(* Logix 5000 AddOnInstructionDefinition export MHSI_Yaskawa; software revision 17.00 *)

TYPE Yaskawa_EIP_Servo :   // Yaskawa SigmaLogic Axis Structure v2.4.0
STRUCT
   O : Yaskawa_OUT_to_Servo;
   I : Yaskawa_IN_from_Servo;
   AOI_SB : Yaskawa_AOI_Status_Bits;
END_STRUCT
END_TYPE

TYPE Yaskawa_OUT_to_Servo :   // Structure of data sent out to the Yaskawa SigmaLogic controller v2.4.0
STRUCT
   b00_ServoOn : BOOL;   // Servo On
   b01_Stop : BOOL;   // Stops All Current Motion in Progress
   b02_Home : BOOL;   // Start Homing Process
   b03_MoveStart1 : BOOL;   // Start Current Motion
   b06_SuperImpose : BOOL;
   b07_ServoAlarmReset : BOOL;   // Servo Alarm Reset
   b08_ControllerAlarmReset : BOOL;   // SigmaLogic Alarm Reset
   b09_MoveStart2 : BOOL;   // Start Second Motion (Blended Move)
   b10_MoveAbort : BOOL;   // Abort Current Move
   b11_MovePause : BOOL;   // Pause Current Move
   b12_SeqPause : BOOL;   // Indexing Sequence Pause
   b13_SeqResume : BOOL;   // Indexing Sequence Resume
   b14_SeqCancel : BOOL;   // Indexing Sequence Cancel
   b15_AbsEncoderReset : BOOL;   // Absolute Encoder Reset
   b16_SeqStart : BOOL;   // Start Indexing Sequence
   b17_SeqEditSpeed : BOOL;   // Enter Edit Speed
   b18_SeqEditDistance : BOOL;   // Enter Distance Edit
   b19_PLSEnable : BOOL;   // Enable PLS execution
   b20_PLSActivateOutput1 : BOOL;   // Activate PLS output1 switch logic
   b21_PLSActivateOutput2 : BOOL;   // Activate PLS output2 switch logic
   b22_PLSActivateOutput3 : BOOL;   // Activate PLS output3 switch logic
   b23_PLSActivateOutput4 : BOOL;   // Activate PLS output4 switch logic
   b24_SetClock : BOOL;   // Set the remote controller clock with data provided by the PLC
   RebootController : BOOL;
   UseExternalEncoder : BOOL;   // Use External Encoder when executing MAHSP_Yaskawa
   b32_HeatbeatAnswer : BOOL;   // Heartbeat Answer
   BrakeBypassRequest : BOOL;
   SetFwdTorqueLimit : BOOL;
   SetRevTorqueLimit : BOOL;
   TorqueLimit : DINT;
   TorqueRamp : DINT;
   HomeMethod : INT;
   HomeSpeed : DINT;
   HomeAccDec : DINT;   // Home Move Acceleration/Deceleration Rate
   HomeBackOffDistance : DINT;
   HomeCreepSpeed : DINT;
   HomeCreepDistanceLimit : DINT;
   HomeCreepTimeLimit : DINT;
   HomeOffsetDistance : DINT;
   HomeOffsetSpeed : DINT;
   HomePostion : DINT;
   HomeTorque : DINT;
   HomeInputNo : DINT;
   HomeApproachTimeLimit : DINT;
   HomeApproachDistLimit : DINT;
   HomeDirection : INT;
   HomeSwitchMode : INT;
   MoveType : INT;
   MoveDirection : INT;
   MoveAccel1 : DINT;
   MoveAccel2 : DINT;
   MoveDecel1 : DINT;
   MoveDecel2 : DINT;
   MoveSpeed1 : DINT;
   MoveSpeed2 : DINT;
   MoveDistance1 : DINT;
   MoveDistance2 : DINT;
   MovePosition1 : DINT;
   MovePosition2 : DINT;
   RegistrationDistance : DINT;
   GearNumerator : DINT;
   GearDenominator : DINT;
   SuperImposeDistance : DINT;
   Resolution : INT;
   RegistrationDirection : INT;
   TuningLevel : INT;
   SequenceStep : INT;   // Staring Sequence Step Number
   SequenceEditStep : INT;   // Sequence Step Number to Edit
   FlagCommandBits1 : DINT;   // Flag Commands. 1..64 are General Flags, Bits 0..31 correspond to Flag 1..32
   FlagCommandBits2 : DINT;   // Flag Commands cont. 1..64 are General Flags, Bits 0..31 correspond to Flag 33..64
   DigitalOutCommandBits : DINT;   // Digital Output commands. Bits 0-7 correspond to CN13 Digital Outputs 0-7, used as Flag 73-80. Bits 8-10 correspond to CN1 Digital Outputs 0-2 used as Flag 88-90"
   SequenceEditSpeed : DINT;
   SequenceEditDistance : DINT;
   FeedRateOverride : INT;
   HSI_Enable : BOOL;
   HSI_MoveMode : BOOL;   // 0=Relative; 1=Moves per Cycle
   HSI_CalcMethod : BOOL;   // 0=Accel/Decel; 1=Time
   HSI_MoveDirection : BOOL;   // 0 = Negative; 1 = Positive
   HSI_TriggerFlag : INT;
   HSI_MovingFlag : INT;
   HSI_DwellingFlag : INT;
   HSI_DoneFlag : INT;
   HSI_MoveType : INT;   // 0=Single; 1=Repeat; 2=Repeat "x" times
   HSI_RepeatNumber : INT;
   HSI_Distance : DINT;
   HSI_Speed : DINT;
   HSI_Accel : DINT;
   HSI_MoveTime : DINT;
   HSI_DwellTime : DINT;
   PLS_OutputFlag1 : INT;
   PLS_OutputFlag2 : INT;
   PLS_OutputFlag3 : INT;
   PLS_OutputFlag4 : INT;
   PLS_OnPosition1 : DINT;
   PLS_OffPosition1 : DINT;
   PLS_OnPosition2 : DINT;
   PLS_OffPosition2 : DINT;
   PLS_OnPosition3 : DINT;
   PLS_OffPosition3 : DINT;
   PLS_OnPosition4 : DINT;
   PLS_OffPosition4 : DINT;
   PLS_OnCompensation1 : INT;
   PLS_OffCompensation1 : INT;
   PLS_OnCompensation2 : INT;
   PLS_OffCompensation2 : INT;
   PLS_OnCompensation3 : INT;
   PLS_OffCompensation3 : INT;
   PLS_OnCompensation4 : INT;
   PLS_OffCompensation4 : INT;
   RTC_Year : INT;
   RTC_Month : INT;
   RTC_Day : INT;
   RTC_Hour : INT;
   RTC_Min : INT;
   RTC_Sec : INT;
   StopDecel : DINT;
   AnalogOutput : INT;   // CN13, AO_01 [mV]
END_STRUCT
END_TYPE

TYPE Yaskawa_AOI_Status_Bits :   // Internal bits used to interlock Yaskawa AOI execution. v2.4.0
STRUCT
   MAM : BOOL;   // Move AOI Active
   MAJ : BOOL;   // Jog AOI Active
   MAB : BOOL;   // Blending AOI Active
   MAG : BOOL;   // Gearing AOI Active
   MAHSP : BOOL;   // Home SetPoint AOI Active
   MAH : BOOL;   // Homing AOI Active
   MSQE : BOOL;   // Sequence Edit AOI Active
   MSQR : BOOL;   // Sequence Run AOI Active
   MHSI : BOOL;   // High Speed Index AOI Active
   MSO : BOOL;   // Servo On
   MSF : BOOL;   // Servo Off
   MAFR : BOOL;   // Fault Reset
   MAS : BOOL;   // Servo Abort
   MTRQ : BOOL;   // Torque Mode Active
   MPLS : BOOL;   // PLS Active
   MCLK : BOOL;   // SetClock Active
   MSTL : BOOL;   // Set Torque Limit Active
   AOI_Permissive : BOOL;   // Permissive to Execute an AOI
END_STRUCT
END_TYPE

TYPE Yaskawa_IN_from_Servo :   // Structure of data coming from the Yaskawa SigmaLogic controller. v2.4.0
STRUCT
   AlarmText : STRING;   // ServoPack Alarm Code plus Text Description
   b00_Heartbeat : BOOL;
   b01_Alarm : BOOL;   // ServoPack Alarm
   b02_Warning : BOOL;   // ServoPack Warning
   b03_Ready : BOOL;   // ServoPack Ready
   b04_Enabled : BOOL;   // ServoPack Enabled ("Servo On")
   b05_StopComplete : BOOL;
   b06_HomeComplete : BOOL;
   b07_HomeBusy : BOOL;
   b08_HomeActive : BOOL;
   b09_HomeAborted : BOOL;
   b10_HomeError : BOOL;
   b11_MoveAbsComplete : BOOL;
   b12_MoveAbsBusy : BOOL;
   b13_MoveAbsActive : BOOL;
   b14_MoveAbsAborted : BOOL;
   b15_MoveAbsError : BOOL;
   b16_MoveRelComplete : BOOL;
   b17_MoveRelBusy : BOOL;
   b18_MoveRelActive : BOOL;
   b19_MoveRelAborted : BOOL;
   b20_MoveRelError : BOOL;
   b21_JogAtSpeed : BOOL;
   b22_JogBusy : BOOL;
   b23_JogActive : BOOL;
   b24_JogAborted : BOOL;
   b25_JogError : BOOL;
   b26_GearInSync : BOOL;
   b27_GearBusy : BOOL;
   b28_GearActive : BOOL;
   b29_GearAborted : BOOL;
   b30_GearError : BOOL;
   b32_MoveSuperComplete : BOOL;
   b33_MoveSuperBusy : BOOL;
   b34_MoveSuperActive : BOOL;
   b35_MoveSuperAborted : BOOL;
   b36_MoveSuperError : BOOL;
   b37_PowerCycleRequired : BOOL;
   b38_MoveBlend1Complete : BOOL;
   b39_MoveBlend1Busy : BOOL;
   b40_MoveBlend1Active : BOOL;
   b41_MoveBlend1Abort : BOOL;
   b42_MoveBlend1Error : BOOL;
   b43_MoveBlend2Complete : BOOL;
   b44_MoveBlend2Busy : BOOL;
   b45_MoveBlend2Active : BOOL;
   b46_MoveBlend2Abort : BOOL;
   b47_MoveBlend2Error : BOOL;
   b48_RegComplete : BOOL;
   b49_RegBusy : BOOL;
   b50_RegActive : BOOL;
   b51_RegAborted : BOOL;
   b52_RegError : BOOL;
   b53_ResetAbsEncoderActive : BOOL;
   b54_ResetAbsEncoderBusy : BOOL;
   b55_ResetAbsEncoderDone : BOOL;
   b56_ResetAbsEncoderError : BOOL;
   b57_SeqRunning : BOOL;
   b58_RegSensorNotReached : BOOL;
   b59_SeqEditError : BOOL;
   b60_SeqEditDone : BOOL;
   b61_TorqueAtTorque : BOOL;
   b62_TorqueBusy : BOOL;
   b63_TorqueActive : BOOL;
   b64_TorqueAborted : BOOL;
   b65_TorqueError : BOOL;
   b66_ControllerAlarm : BOOL;
   b67_ApplicationError : BOOL;
   b68_AxisAtStandStill : BOOL;
   b69_TestModeActive : BOOL;
   b70_ServoParamsOK : BOOL;
   b71_SetFwdTorqueLimitDone : BOOL;
   b72_SetRevTorqueLimitDone : BOOL;
   Position : DINT;
   Speed : DINT;
   Torque : DINT;
   HomeErrorID : INT;
   MoveAbsErrorID : INT;
   MoveRelErrorID : INT;
   JogErrorID : INT;
   GearErrorID : INT;
   MoveSuperErrorID : INT;
   ServoAlarmID : INT;
   ServoWarningID : INT;
   ControllerAlarmID : DINT;
   AxisGenAlarmID : DINT;
   MoveBlend1ErrorID : INT;
   MoveBlend2ErrorID : INT;
   ResetAbsEncoderErrorID : INT;
   FunctionBlockErrorID : INT;
   TorqueErrorID : INT;
   RegErrorID : INT;
   SeqCurrentStep : INT;
   FlagStatusBit1 : DINT;   // Flag Status. 1..64 are General Flags, Bits 0..31 correspond to Flag 1..32
   FlagStatusBit2 : DINT;   // Flag Status cont. 1..64 are General Flags, Bits 0..31 correspond to Flag 33..64
   IOStatusBits : DINT;   // Digital IO Status. Bits 0-7, CN13 Inputs 0-7, Used as Flag 65-72. Bits 8-15, CN13 Outputs 0-7, Used as Flag 73-80. Bits 16-22, CN1 Inputs 0-6, Used as Flag 81-87. Bits 23-25, CN1 Outputs 0-4, Used as Flag 88-92.
   HSI_Moving : BOOL;
   HSI_Dwelling : BOOL;
   HSI_Done : BOOL;
   HSI_Busy : BOOL;
   HSI_Error : BOOL;
   HSI_ErrorCode : INT;
   PLS_Running : BOOL;
   PLS_SwitchStatus1 : BOOL;
   PLS_SwitchStatus2 : BOOL;
   PLS_SwitchStatus3 : BOOL;
   PLS_SwitchStatus4 : BOOL;
   PLS_Busy : BOOL;
   PLS_Error : BOOL;
   PLS_ErrorCode : INT;
   SetClock_Done : BOOL;
   SetClock_Busy : BOOL;
   SetClock_Error : BOOL;
   SetClock_ErrorID : INT;
   SoftwareVersion : DINT;
   FirmwareVersion : DINT;
   CommandedPos : DINT;
   CommandedPosNonCyc : DINT;
   CommandedSpeed : DINT;
   Clock_Year : INT;
   Clock_Month : INT;
   Clock_Day : INT;
   Clock_Hour : INT;
   Clock_Minute : INT;
   Clock_Second : INT;
   AnalogInput : REAL;   // CN13, AI_01 [v]
   BrakeBypassActive : BOOL;
   ForwardTorqueLimit : DINT;
   ReverseTorqueLimit : DINT;
END_STRUCT
END_TYPE

ADD_ON_INSTRUCTION MHSI_Yaskawa   (* revision 2.4 0, vendor Yaskawa America, Inc., ExecuteEnableInFalse *)
// Motion Axis High Speed Index
// Revision note:
// 2.4.0: No functional change
// 2.3.1: Moved unlatch of AOI_ON_LOCAL to bottom of EnableInFalse routine so that outputs will be on for at least 1 scan if one-shot on EN is used.
// 2.3.0: No functional change
// 2.0.0: Improved output operation and error code reporting. Improved interlocking with embedded code.
// 1.2.0: No functional change.
// Initial Release 9/10/2014
// Help:
// This AOI transfers settings to the remote axis node for high response motion to be executed in the remote node using local servo I/O. The motion goes through a Move-Dwell cycle when triggered. Move time can either be entered directly or derived from the Speed, Accel and Distance parameters.
VAR_IN_OUT
   Axis : Yaskawa_EIP_Servo; {required}
END_VAR
VAR_INPUT
   MoveMode : INT; {required}   // 0 = Relative 1 = Moves per Machine Cycle
   MoveType : INT; {required}   // 0 = Single 1 = Repeating Move 2 = Repeat for "x" Times
   RepeatNumber : INT; {required}   // For MoveType #2
   CalcMethod : INT; {required}   // 0 = Use Acc/ Decel 1 = Use Time
   Distance : REAL; {required}   // [units]
   Speed : REAL; {required}   // [units/s]
   Accel : REAL; {required}   // [units/s/s]
   MoveTime : DINT; {required}   // msec
   DwellTime : DINT; {required}   // msec
   Direction : INT; {required}   // 0 = Positive 1 = Negative
   TriggerFlagAssign : INT; {required}
   MovingFlagAssign : INT; {required}
   DwellingFlagAssign : INT; {required}
   DoneFlagAssign : INT; {required}
END_VAR
VAR_OUTPUT
   EN : BOOL; {visible}   // AOI is Active
   DN : BOOL; {visible}   // HSI Cycle (Index then Dwell) Completed
   IP : BOOL; {visible}   // HSI Busy (move in operation)
   ER : BOOL; {visible}   // HSI Error
   MV : BOOL; {visible}   // HSI Move (move is in motion)
   DW : BOOL; {visible}   // HSI Dwelling
   FLT_RDY : BOOL; {visible}   // The Servo is Not Ready
   FLT_BSY : BOOL; {visible}   // There is another AOI Active for this Axis
   ErrorCode : INT; {visible}   // ErrorID for High Speed Index function
END_VAR
VAR
   AOI_ON_LOCAL : BOOL;
   ScaleFactor : DINT;
   Finished : BOOL;   // Function is Finished
END_VAR

ROUTINE EnableInFalse   (* ladder *)
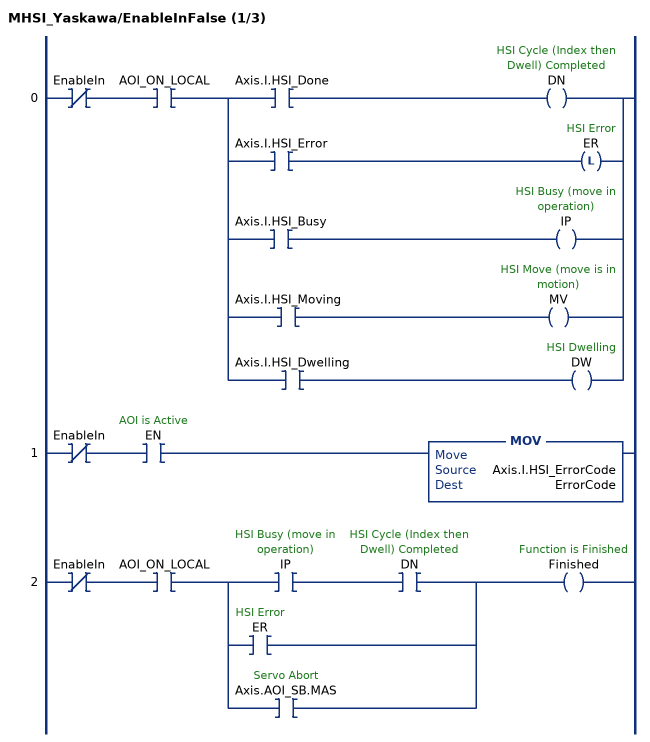
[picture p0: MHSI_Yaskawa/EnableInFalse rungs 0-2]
   0: XIO(EnableIn)XIC(AOI_ON_LOCAL)[XIC(Axis.I.HSI_Done) OTE(DN) ,XIC(Axis.I.HSI_Error) OTL(ER) ,XIC(Axis.I.HSI_Busy) OTE(IP) ,XIC(Axis.I.HSI_Moving) OTE(MV) ,XIC(Axis.I.HSI_Dwelling) OTE(DW) ];
   1: XIO(EnableIn)XIC(EN)MOV(Axis.I.HSI_ErrorCode,ErrorCode);
   2: XIO(EnableIn)XIC(AOI_ON_LOCAL)[XIC(IP) XIC(DN) ,XIC(ER) ,XIC(Axis.AOI_SB.MAS) ]OTE(Finished);
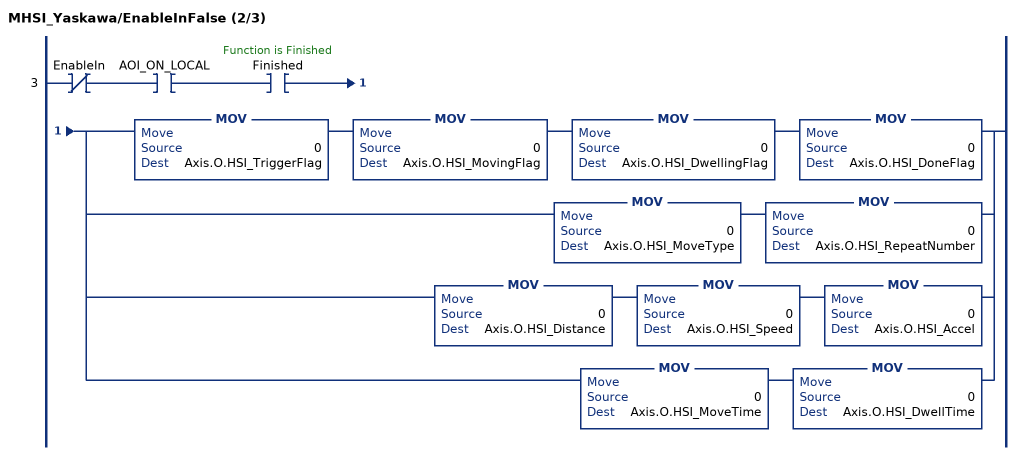
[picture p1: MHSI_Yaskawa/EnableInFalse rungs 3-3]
   3: XIO(EnableIn)XIC(AOI_ON_LOCAL)XIC(Finished)[MOV(0,Axis.O.HSI_TriggerFlag) MOV(0,Axis.O.HSI_MovingFlag) MOV(0,Axis.O.HSI_DwellingFlag) MOV(0,Axis.O.HSI_DoneFlag) ,MOV(0,Axis.O.HSI_MoveType) MOV(0,Axis.O.HSI_RepeatNumber) ,MOV(0,Axis.O.HSI_Distance) MOV(0,Axis.O.HSI_Speed) MOV(0,Axis.O.HSI_Accel) ,MOV(0,Axis.O.HSI_MoveTime) MOV(0,Axis.O.HSI_DwellTime) ];
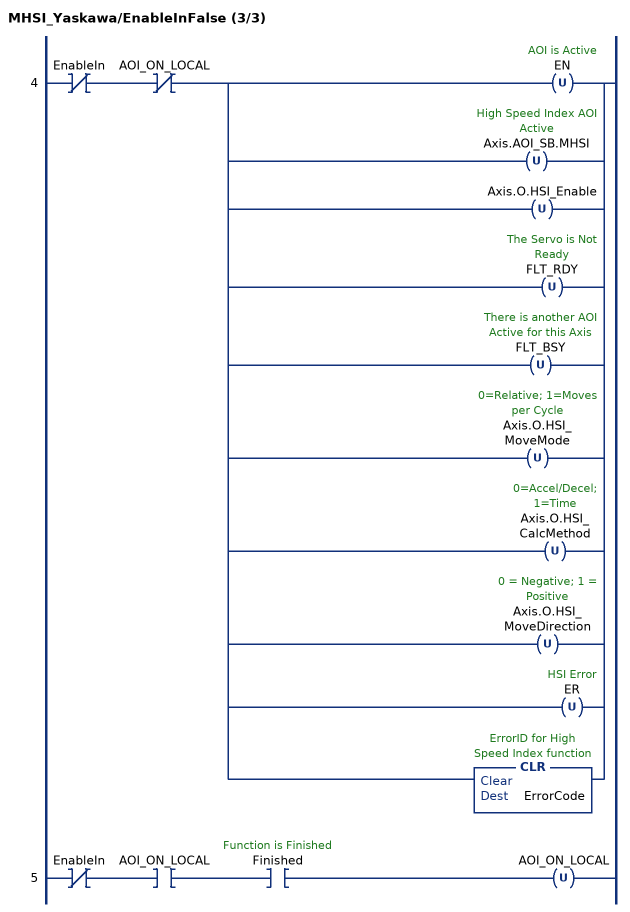
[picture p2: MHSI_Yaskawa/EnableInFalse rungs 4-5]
   4: XIO(EnableIn)XIO(AOI_ON_LOCAL)[OTU(EN) ,OTU(Axis.AOI_SB.MHSI) ,OTU(Axis.O.HSI_Enable) ,OTU(FLT_RDY) ,OTU(FLT_BSY) ,OTU(Axis.O.HSI_MoveMode) ,OTU(Axis.O.HSI_CalcMethod) ,OTU(Axis.O.HSI_MoveDirection) ,OTU(ER) ,CLR(ErrorCode) ];
   5: XIO(EnableIn)XIC(AOI_ON_LOCAL)XIC(Finished)OTU(AOI_ON_LOCAL);
END_ROUTINE

ROUTINE Logic   (* ladder *)
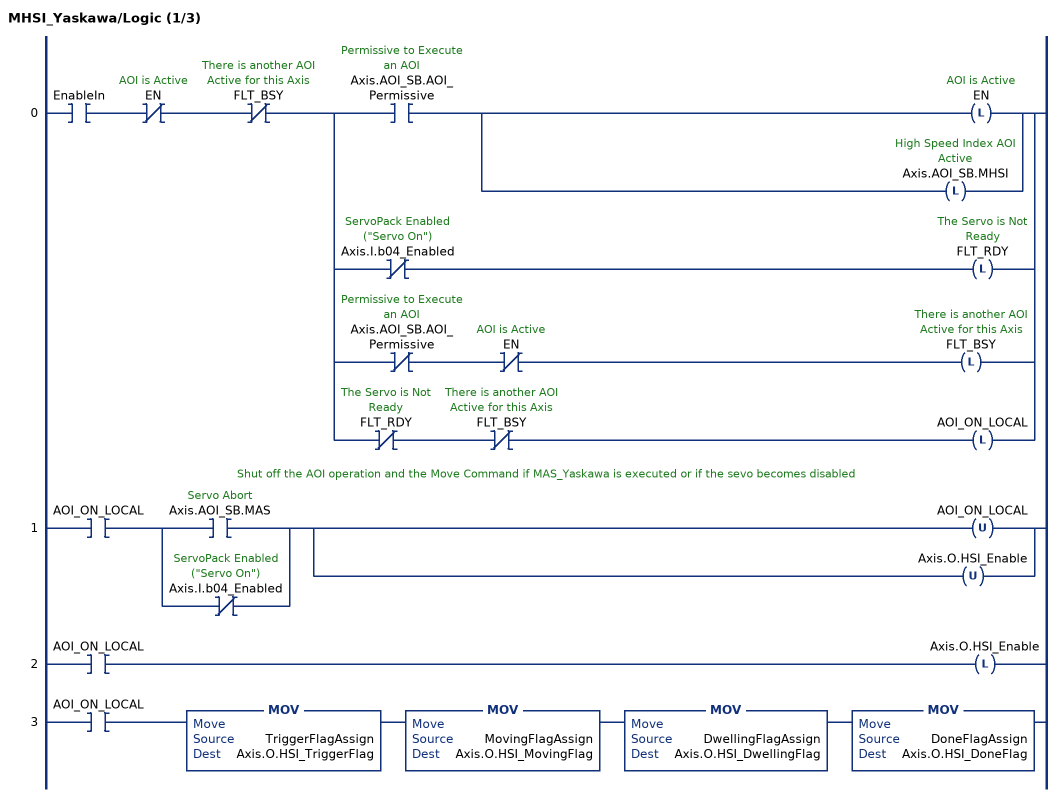
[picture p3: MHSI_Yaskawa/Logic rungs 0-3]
   0: XIC(EnableIn)XIO(EN)XIO(FLT_BSY)[XIC(Axis.AOI_SB.AOI_Permissive) [OTL(EN) ,OTL(Axis.AOI_SB.MHSI) ] ,XIO(Axis.I.b04_Enabled) OTL(FLT_RDY) ,XIO(Axis.AOI_SB.AOI_Permissive) XIO(EN) OTL(FLT_BSY) ,XIO(FLT_RDY) XIO(FLT_BSY) OTL(AOI_ON_LOCAL) ];
   // Shut off the AOI operation and the Move Command if MAS_Yaskawa is executed or if the sevo becomes disabled
   1: XIC(AOI_ON_LOCAL)[XIC(Axis.AOI_SB.MAS) ,XIO(Axis.I.b04_Enabled) ][OTU(AOI_ON_LOCAL) ,OTU(Axis.O.HSI_Enable) ];
   2: XIC(AOI_ON_LOCAL)OTL(Axis.O.HSI_Enable);
   3: XIC(AOI_ON_LOCAL)MOV(TriggerFlagAssign,Axis.O.HSI_TriggerFlag)MOV(MovingFlagAssign,Axis.O.HSI_MovingFlag)MOV(DwellingFlagAssign,Axis.O.HSI_DwellingFlag)MOV(DoneFlagAssign,Axis.O.HSI_DoneFlag);
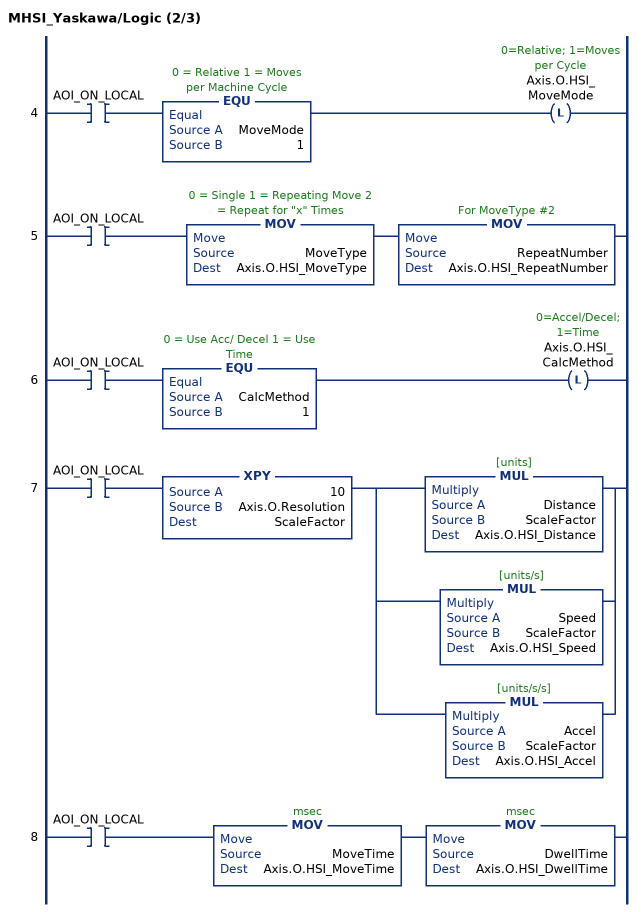
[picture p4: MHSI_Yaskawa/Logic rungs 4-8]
   4: XIC(AOI_ON_LOCAL)EQU(MoveMode,1)OTL(Axis.O.HSI_MoveMode);
   5: XIC(AOI_ON_LOCAL)MOV(MoveType,Axis.O.HSI_MoveType)MOV(RepeatNumber,Axis.O.HSI_RepeatNumber);
   6: XIC(AOI_ON_LOCAL)EQU(CalcMethod,1)OTL(Axis.O.HSI_CalcMethod);
   7: XIC(AOI_ON_LOCAL)XPY(10,Axis.O.Resolution,ScaleFactor)[MUL(Distance,ScaleFactor,Axis.O.HSI_Distance) ,MUL(Speed,ScaleFactor,Axis.O.HSI_Speed) ,MUL(Accel,ScaleFactor,Axis.O.HSI_Accel) ];
   8: XIC(AOI_ON_LOCAL)MOV(MoveTime,Axis.O.HSI_MoveTime)MOV(DwellTime,Axis.O.HSI_DwellTime);
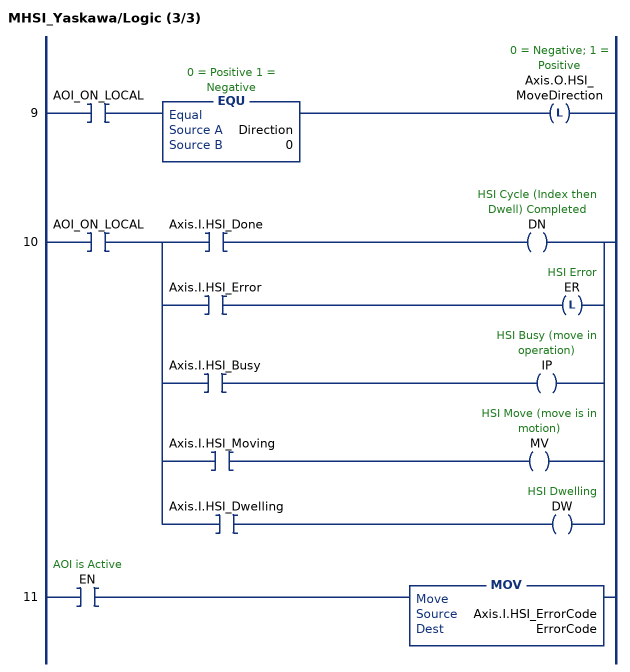
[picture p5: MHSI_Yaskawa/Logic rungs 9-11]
   9: XIC(AOI_ON_LOCAL)EQU(Direction,0)OTL(Axis.O.HSI_MoveDirection);
   10: XIC(AOI_ON_LOCAL)[XIC(Axis.I.HSI_Done) OTE(DN) ,XIC(Axis.I.HSI_Error) OTL(ER) ,XIC(Axis.I.HSI_Busy) OTE(IP) ,XIC(Axis.I.HSI_Moving) OTE(MV) ,XIC(Axis.I.HSI_Dwelling) OTE(DW) ];
   11: XIC(EN)MOV(Axis.I.HSI_ErrorCode,ErrorCode);
END_ROUTINE
END_ADD_ON_INSTRUCTION
